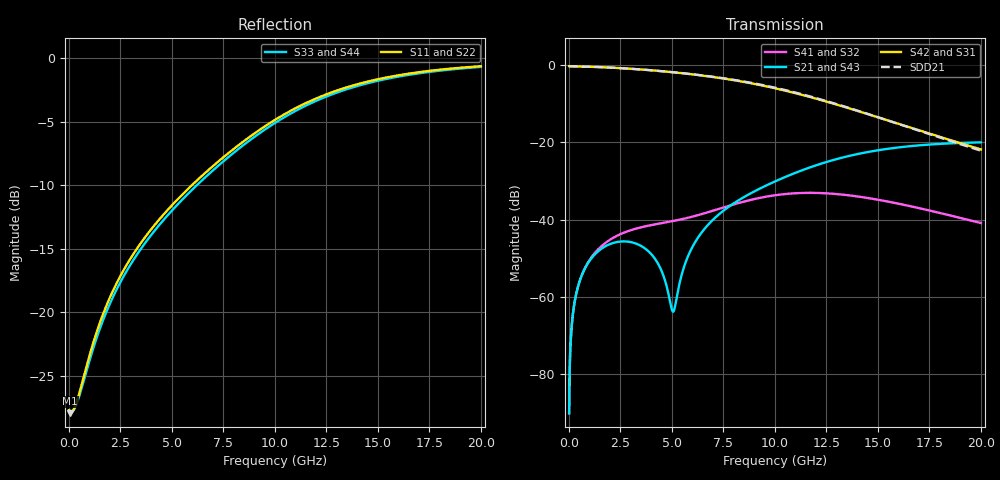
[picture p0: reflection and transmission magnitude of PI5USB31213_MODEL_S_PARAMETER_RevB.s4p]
! NPort=4 DATA=800 NOISE=0 GROUPDELAY=0 COMPLEX_DATAFORMAT=POLAR
! NumOfBlock=1 NumOfParam=0
! .MODEL Smodel S TSTONEFILE=PI5USB31213_4PORT_S_PARAMETER_RevB.s4p TYPE=S
!  -- The above .MODEL line can be used for the S element in the netlist.
!PORT1 = INPUT+
!PORT2 = INPUT-
!PORT3 = OUTPUT+
!PORT4 = OUTPUT-
# Hz S MA R  50
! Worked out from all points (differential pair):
!   800 points, 10 MHz to 20 GHz, reference 50 ohm
!   strongest paths, dB at 10 MHz, 5.014 GHz, 10.02 GHz, 15.02 GHz, 20 GHz:
!     S42: -0.4, -1.9, -6.1, -13.6, -21.9
!     S31: -0.4, -1.9, -6.1, -13.6, -21.9
!     S21: -90.0, -63.5, -30.1, -22.1, -20.1
!     S43: -90.0, -65.8, -30.1, -22.2, -20.1
!     S41: -90.1, -40.4, -33.7, -34.9, -40.9
!     S32: -90.1, -40.4, -33.7, -34.9, -40.9
!   taken as a pair (ports 2,1 in; 4,3 out), SDD21 dB: -0.4, -1.9, -5.9, -13.6, -22.2
!   lowest |S11| = -27.9 dB at 60.04 MHz (marker M1), VSWR 1.08, Z = 54.1 - j0.604 ohm
!   |S11| at or under -10 dB: start of sweep to 5.968 GHz
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1e7  0.04127 -1.9  3.146e-05 89.7  0.9583 -0.2  3.135e-05 89.7
     3.146e-05 89.7  0.04127 -1.9  3.135e-05 89.7  0.9583 -0.2
     0.9583 -0.2  3.135e-05 89.7  0.04127 -1.9  3.146e-05 89.7
     3.135e-05 89.7  0.9583 -0.2  3.146e-05 89.7  0.04127 -1.9
6.00375e7  0.04014 -8.0  0.0001882 88.6  0.9563 -1.2  0.0001875 88.5
           0.0001882 88.6  0.04014 -8.0  0.0001875 88.5  0.9563 -1.2
           0.9563 -1.2  0.0001875 88.5  0.04012 -7.7  0.0001882 88.6
           0.0001875 88.5  0.9563 -1.2  0.0001882 88.6  0.04012 -7.7
8.3562e8  0.06055 -73.2  0.002488 73.0  0.9455 -14.6  0.00253 72.2
          0.002488 73.0  0.06055 -73.2  0.00253 72.2  0.9455 -14.6
          0.9456 -14.5  0.002531 72.3  0.0582 -71.6  0.002488 73.2
          0.002531 72.3  0.9456 -14.5  0.002488 73.2  0.0582 -71.6
3.06229e9  0.1664 -148.9  0.005067 30.6  0.884 -52.3  0.007358 32.2
           0.005067 30.6  0.1664 -148.9  0.007358 32.2  0.884 -52.3
           0.8851 -51.9  0.007367 32.6  0.1576 -149.1  0.00507 31.5
           0.007367 32.6  0.8851 -51.9  0.00507 31.5  0.1576 -149.1
5.06379e9  0.267 164.6  0.0006443 -86.9  0.7967 -85.4  0.009538 10.1
           0.0006443 -86.9  0.267 164.6  0.009538 10.1  0.7967 -85.4
           0.7993 -84.7  0.009569 10.8  0.2547 163.5  0.000488 -89.4
           0.009569 10.8  0.7993 -84.7  0.000488 -89.4  0.2547 163.5
8.5414e9  0.4746 94.7  0.01981 148.0  0.5914 -142.3  0.01704 -26.5
          0.01981 148.0  0.4746 94.7  0.01704 -26.5  0.5914 -142.3
          0.5964 -141.3  0.01718 -25.5  0.4595 93.4  0.01989 146.5
          0.01718 -25.5  0.5964 -141.3  0.01989 146.5  0.4595 93.4
2e10  0.9293 -45.8  0.09933 45.8  0.07849 86.8  0.00879 154.5
      0.09933 45.8  0.9293 -45.8  0.00879 154.5  0.07849 86.8
      0.08053 88.0  0.009019 155.7  0.9234 -45.9  0.09861 45.8
      0.009019 155.7  0.08053 88.0  0.09861 45.8  0.9234 -45.9
